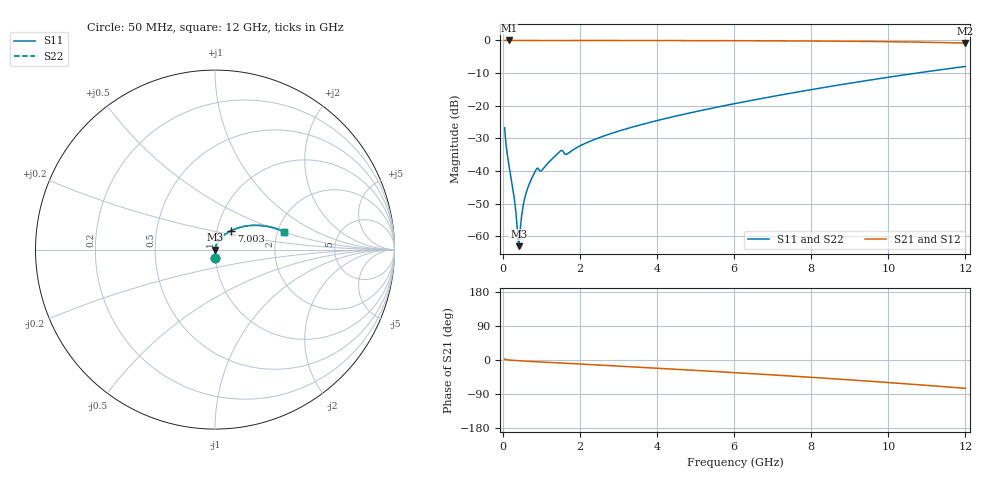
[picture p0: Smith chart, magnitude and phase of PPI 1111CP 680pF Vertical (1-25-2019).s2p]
# GHz S MA R 50
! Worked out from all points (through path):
!   1601 points, 50 MHz to 12 GHz, reference 50 ohm
!   highest |S21| = 0.00 dB at 162 MHz (marker M1); lowest = -0.8 dB at 12 GHz (marker M2)
!   group delay of S21, straight-line fit = 17.1 ps
!   lowest |S11| = -63.0 dB at 416 MHz (marker M3), VSWR 1.00, Z = 50.1 - j0.00309 ohm
!   |S11| at or under -10 dB: start of sweep to 10.74 GHz
!   |S22| runs from -63.0 to -8.0 dB; largest |S21 - S12| = 0
!   S11 on the Smith chart (normalised r, x): 50 MHz: 1.00, -0.09; 7.003 GHz: 1.17, +0.25; 12 GHz: 2.18, +0.52
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0.05  0.04605 -87.2  0.9986 2.4  0.9986 2.4  0.04605 -87.2
0.08734375  0.0256 -88.1  0.9993 1.1  0.9993 1.1  0.0256 -88.1
0.1620312  0.01227 -87.8  0.9994 -0.0  0.9994 -0.0  0.01227 -87.8
0.289  0.004258 -83.0  0.9994 -1.1  0.9994 -1.1  0.004258 -83.0
0.378625  0.001271 -59.6  0.9993 -1.7  0.9993 -1.7  0.001271 -59.6
0.4159687  0.0007042 -2.5  0.9993 -1.9  0.9993 -1.9  0.0007042 -2.5
0.4533125  0.00122 50.9  0.9992 -2.2  0.9992 -2.2  0.00122 50.9
0.528  0.002875 71.4  0.9992 -2.6  0.9992 -2.6  0.002875 71.4
0.6026875  0.004489 76.0  0.9991 -3.0  0.9991 -3.0  0.004489 76.0
0.70725  0.006698 77.8  0.9989 -3.7  0.9989 -3.7  0.006698 77.8
0.856625  0.01024 74.1  0.9979 -4.5  0.9979 -4.5  0.01024 74.1
1.020938  0.01031 72.1  0.9976 -5.3  0.9976 -5.3  0.01031 72.1
1.491469  0.02016 71.9  0.9962 -8.0  0.9962 -8.0  0.02016 71.9
1.670719  0.01819 70.3  0.9963 -8.7  0.9963 -8.7  0.01819 70.3
2.044156  0.02489 75.2  0.9978 -10.9  0.9978 -10.9  0.02489 75.2
2.85825  0.03825 72.0  0.9973 -15.3  0.9973 -15.3  0.03825 72.0
4.038312  0.05989 66.1  0.9959 -21.9  0.9959 -21.9  0.05989 66.1
6.025  0.1078 55.2  0.9912 -33.4  0.9912 -33.4  0.1078 55.2
7.003406  0.1387 49.4  0.9869 -39.3  0.9869 -39.3  0.1387 49.4
8.019156  0.177 43.1  0.9804 -45.8  0.9804 -45.8  0.177 43.1
10.01331  0.2737 29.6  0.9571 -59.5  0.9571 -59.5  0.2737 29.6
12  0.3995 14.4  0.9108 -74.8  0.9108 -74.8  0.3995 14.4
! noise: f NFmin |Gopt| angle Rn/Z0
0.05  0.0003806  0.8688  0.2577  0.0006243
1.372  0.00488  0.7394  6.295  0.003739
2.701  0.006765  0.6511  12.24  0.003646
4.031  0.009015  0.6209  18.03  0.004335
5.36  0.01125  0.606  23.64  0.005071
6.682  0.0135  0.6  29.02  0.00585
8.012  0.01584  0.6007  34.21  0.00672
9.341  0.01834  0.607  39.19  0.007721
10.67  0.02106  0.618  43.97  0.00891
12  0.02408  0.6331  48.55  0.01036
